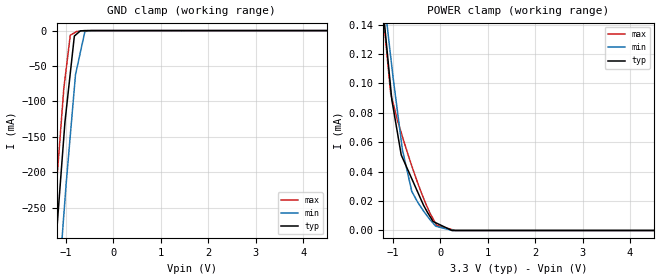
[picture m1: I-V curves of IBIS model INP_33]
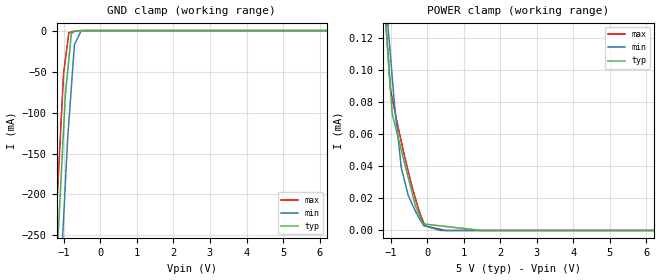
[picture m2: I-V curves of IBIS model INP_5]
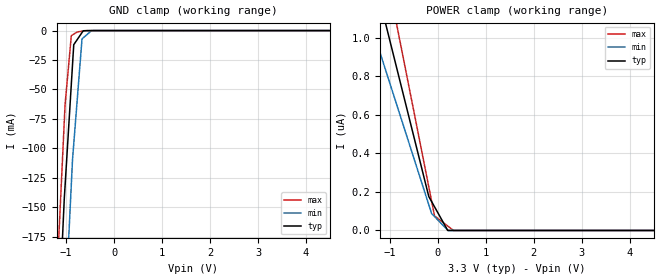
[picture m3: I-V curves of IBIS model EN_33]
| Texas Instruments Incorporated
| 6KVpeak Low Power Triple and Quad Channels Digital Isolators
| 25 Mbps (C) and 150 Mbps (M) speed grades.
| Marketing part#   Voltage Range   Package-type   #pins/pkg drawing
| ISO7640FMDW   3V - 5.5V   SOIC   16-pin DW
| ISO7640FMDWR   3V - 5.5V   SOIC   16-pin DW
| ISO7640FCDW   3V - 5.5V   SOIC   16-pin DW
| ISO7640FCDWR   3V - 5.5V   SOIC   16-pin DW
| ISO7641FMDW   3V - 5.5V   SOIC   16-pin DW
| ISO7641FMDWR   3V - 5.5V   SOIC   16-pin DW
| ISO7641FCDW   3V - 5.5V   SOIC   16-pin DW
| ISO7641FCDWR   3V - 5.5V   SOIC   16-pin DW
| ISO7631FMDW   3V - 5.5V   SOIC   16-pin DW
| ISO7631FMDWR   3V - 5.5V   SOIC   16-pin DW
| ISO7631FCDW   3V - 5.5V   SOIC   16-pin DW
| ISO7631FCDWR   3V - 5.5V   SOIC   16-pin DW
[IBIS Ver]   4.0
[File name]   iso75xx.ibs
[File Rev]   1.1
[Date]   03/13/2012
[Source]   Model built from TISPICED simulations at:
   Texas Instruments Incorporated.
   Analog-eLab, HPA
   12500 TI Blvd
   Dallas, TX -75243
   For Support e-mail: elab_ibis@list.ti.com
[Notes]   Revision History
   Rev 1.0: 6/13/2011
   Rev 1.1: 3/13/2012 Added 25 Mbps speed grade output buffer
   - Pulldown/up in OUTM/OUTC non-monotonic warnings reflect true buffer behavior
   - C_comp although listed in numberical order of value are obtained from varying PVT conditions.
   For PVT conditions for each specific value, refer to the buffer description under repective [Model].
   IBIS model user is responsible for using appropriate C_comp to simulate for Signal Integrity.
[Disclaimer] This model is designed as an aid for customers of Texas Instruments.
 TI and its licensors and suppliers make no warranties, either expressed
 or implied, with respect to this  model, including the warranties of
 merchantability or fitness for a particular purpose.
 The model is provided solely on an "as is" basis. The entire risk as to
 its quality and performance is with the customer.
[Copyright] (C)Copyright 2012 Texas Instruments Incorporated.
   All rights reserved.
|   Component ISO7640F
[Component]   ISO7640F
[Manufacturer]  Texas Instruments Incorporated
[Package]   |16-pin SOIC DW package
|   typ   min   max
R_pkg   0.10903   0.02188   0.19738
L_pkg   1.81763nH   0.55719nH   2.72701nH
C_pkg   0.46541pF   0.23901pF   0.75876pF
[Pin] signal_name   model_name   R_pin   L_pin   C_pin
   1  VCC1   POWER   0.10139   2.72701n   0.70015p
   2  GND1   GND   0.12533   2.59840n   0.28313p
   3  INA   INP   0.19738   2.59444n   0.23901p
   4  INB   INP   0.12501   1.60826n   0.59739p
   5  INC   INP   0.09868   1.27583n   0.33612p
   6  IND   INP   0.15228   1.98345n   0.42023p
   7  NC   NC   0.02188   0.55719n   0.33803p
   8  GND1   GND   0.09581   2.52990n   0.46538p
   9  GND2   GND   0.10168   2.16452n   0.38933p
   10  EN   EN   0.16987   2.23387n   0.49303p
   11  OUTD   OUT   0.14297   1.85926n   0.49369p
   12  OUTC   OUT   0.10283   1.32835n   0.29474p
   13  OUTB   OUT   0.07399   1.10755n   0.43265p
   14  OUTA   OUT   0.08416   1.26268n   0.45009p
   15  GND2   GND   0.06629   1.45518n   0.75876p
   16  VCC2   POWER   0.08496   1.80603n   0.75490p
[Pin Mapping]pulldown_ref pullup_ref gnd_clamp_ref power_clamp_ref |ext_ref
1   NC   PWRBUS1  |VCC1
2   GNDBUS1   NC   |GND1
3   NC   NC   GNDBUS1   PWRBUS1
4   NC   NC   GNDBUS1   PWRBUS1
5   NC   NC   GNDBUS1   PWRBUS1
6   NC   NC   GNDBUS1   PWRBUS1
7   NC   NC
8   GNDBUS1   NC   |GND1
9   GNDBUS2   NC   |GND2
10   NC   NC   GNDBUS2   PWRBUS2
11   GNDBUS2   PWRBUS2   GNDBUS2   PWRBUS2
12   GNDBUS2   PWRBUS2   GNDBUS2   PWRBUS2
13   GNDBUS2   PWRBUS2   GNDBUS2   PWRBUS2
14   GNDBUS2   PWRBUS2   GNDBUS2   PWRBUS2
15   GNDBUS2   NC   |GND2
16   NC   PWRBUS2  |VCC2
|   Component ISO7641F
[Component]   ISO7641F
[Manufacturer]  Texas Instruments Incorporated
[Package]   |16-pin SOIC DW package
|   typ   min   max
R_pkg   0.10681   0.06298   0.16885
L_pkg   1.70911nH   1.15087nH   2.22009nH
C_pkg   0.45120pF   0.20111pF   0.73257pF
[Pin] signal_name   model_name   R_pin   L_pin   C_pin
   1  VCC1   POWER   0.08793   2.21738n   0.66791p
   2  GND1   GND   0.10467   2.09455n   0.25132p
   3  INA   INP   0.13798   1.78864n   0.20111p
   4  INB   INP   0.09011   1.16823n   0.57349p
   5  INC   INP   0.10921   1.41023n   0.34068p
   6  OUTD   OUT   0.14555   1.89355n   0.41488p
   7  EN1   EN   0.16885   2.22009n   0.43190p
   8  GND1   GND   0.08161   2.08117n   0.43691p
   9  GND2   GND   0.07697   1.92728n   0.40234p
   10  EN2   EN   0.15712   2.06097n   0.48728p
   11  IND   INP   0.11312   1.46878n   0.47723p
   12  OUTC   OUT   0.10925   1.41018n   0.29792p
   13  OUTB   OUT   0.10585   1.36324n   0.34974p
   14  OUTA   OUT   0.07689   1.15087n   0.42179p
   15  GND2   GND   0.06298   1.36962n   0.73218p
   16  VCC2   POWER   0.08085   1.72105n   0.73257p
[Pin Mapping]pulldown_ref pullup_ref gnd_clamp_ref power_clamp_ref |ext_ref
1   NC   PWRBUS1  |VCC1
2   GNDBUS1   NC   |GND1
3   NC   NC   GNDBUS1   PWRBUS1
4   NC   NC   GNDBUS1   PWRBUS1
5   NC   NC   GNDBUS1   PWRBUS1
6   GNDBUS1   PWRBUS1   GNDBUS1   PWRBUS1
7   NC   NC   GNDBUS1   PWRBUS1
8   GNDBUS1   NC   |GND1
9   GNDBUS2   NC   |GND2
10   NC   NC   GNDBUS2   PWRBUS2
11   NC   NC   GNDBUS2   PWRBUS2
12   GNDBUS2   PWRBUS2   GNDBUS2   PWRBUS2
13   GNDBUS2   PWRBUS2   GNDBUS2   PWRBUS2
14   GNDBUS2   PWRBUS2   GNDBUS2   PWRBUS2
15   GNDBUS2   NC   |GND2
16   NC   PWRBUS2  |VCC2
|   Component ISO7631F
[Component]   ISO7631F
[Manufacturer]  Texas Instruments Incorporated
[Package]   |16-pin SOIC DW package
|   typ   min   max
R_pkg   0.10681   0.06298   0.16885
L_pkg   1.70911nH   1.15087nH   2.22009nH
C_pkg   0.45120pF   0.20111pF   0.73257pF
[Pin] signal_name   model_name   R_pin   L_pin   C_pin
   1  VCC1   POWER   0.08793   2.21738n   0.66791p
   2  GND1   GND   0.10467   2.09455n   0.25132p
   3  INA   INP   0.13798   1.78864n   0.20111p
   4  INB   INP   0.09011   1.16823n   0.57349p
   5  OUTC   OUT   0.10921   1.41023n   0.34068p
   6  NC   NC   0.14555   1.89355n   0.41488p
   7  EN1   EN   0.16885   2.22009n   0.43190p
   8  GND1   GND   0.08161   2.08117n   0.43691p
   9  GND2   GND   0.07697   1.92728n   0.40234p
   10  EN2   EN   0.15712   2.06097n   0.48728p
   11  NC   NC   0.11312   1.46878n   0.47723p
   12  INC   INP   0.10925   1.41018n   0.29792p
   13  OUTB   OUT   0.10585   1.36324n   0.34974p
   14  OUTA   OUT   0.07689   1.15087n   0.42179p
   15  GND2   GND   0.06298   1.36962n   0.73218p
   16  VCC2   POWER   0.08085   1.72105n   0.73257p
[Pin Mapping]pulldown_ref pullup_ref gnd_clamp_ref power_clamp_ref |ext_ref
1   NC   PWRBUS1  |VCC1
2   GNDBUS1   NC   |GND1
3   NC   NC   GNDBUS1   PWRBUS1
4   NC   NC   GNDBUS1   PWRBUS1
5   GNDBUS1   PWRBUS1   GNDBUS1   PWRBUS1
6   NC   NC   NC   NC
7   NC   NC   GNDBUS1   PWRBUS1
8   GNDBUS1   NC   |GND1
9   GNDBUS2   NC   |GND2
10   NC   NC   GNDBUS2   PWRBUS2
11   NC   NC
12   NC   NC   GNDBUS2   PWRBUS2
13   GNDBUS2   PWRBUS2   GNDBUS2   PWRBUS2
14   GNDBUS2   PWRBUS2   GNDBUS2   PWRBUS2
15   GNDBUS2   NC   |GND2
16   NC   PWRBUS2  |VCC2
[Model Selector] INP
INP_33   INP Input model for 3.0V - 3.6V
INP_5   INP Input model for 4.5V - 5.5V
[Model Selector] EN
EN_33   EN Input model for 3.0V - 3.6V
EN_5   EN Input model for 4.5V - 5.5V
[Model Selector] OUT
OUTM_33   Output model for 3.0V - 3.6V, 150 Mbps max datarate
OUTM_5   Output model for 4.5V - 5.5V, 150 Mbps max datarate
OUTC_33   Output model for 3.0V - 3.6V, 25 Mbps max datarate
OUTC_5   Output model for 4.5V - 5.5V, 25 Mbps max datarate
| Models and submodels in the file (8): INP_33 (Input), INP_5 (Input), EN_33 (Input), EN_5 (Input), OUTM_33 (3-state), OUTM_5 (3-state), OUTC_5 (3-state), OUTC_33 (3-state)
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|   INP_33 Model
[Model]   INP_33
Model_type   Input
Vinl = .8
Vinh = 2
|   typ   min   max
|   (typ PVT)   (Fast PVT)   (Slow PVT)
C_comp   0.4547p   0.3924p   0.5244p
[Voltage Range]   3.3   3   3.6
[Temperature Range]   27   125   -40
[Power Clamp Reference]   3.3   3   3.6
[GND Clamp Reference]   -0   -0   -0
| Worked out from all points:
|   GND clamp passes 1 mA (typ) near -0.71 V on its own axis
[GND Clamp]
|   Voltage   I(typ)   I(min)   I(max)
-3.3V     -2.332A    -2.436A    -2.268A
-1.394V   -467.7mA   -579.5mA   -397.5mA
-1.244V   -327.2mA   -439.7mA   -256.1mA
-1.196V   -283.3mA   -394.7mA   -213.7mA
-1.046V   -150.4mA   -260.4mA   -81.66mA
-909.8mV  -60.2mA    -148.2mA   -6.478mA
-824.2mV  -7.726mA   -81.21mA   -3.179mA
-800mV    -6.326mA   -62.34mA   -2.25mA
-773.4mV  -4.78mA    -54.13mA   -1.224mA
-602mV    -88.69uA   -1.316mA   -137.7uA
-475.9mV  -46.02uA   -55.21uA   -12.29uA
6.6V      0A         0A         0A
[POWER Clamp]
|   Voltage   I(typ)   I(min)   I(max)
-3.3V     952uA      800.7uA    1.137mA
-1.196V   146.8uA    160.4uA    143.7uA
-1.046V   96.81uA    118.1uA    92.98uA
-1.022V   88.8uA     111.4uA    89.92uA
-824.2mV  51.34uA    61.14uA    66.48uA
-800mV    49.59uA    55.12uA    63.91uA
-602mV    35.2uA     26.59uA    43.91uA
-355.6mV  17.3uA     13.32uA    22.1uA
-152.1mV  6.109uA    4.946uA    7.838uA
-97.62mV  5.269uA    2.928uA    4.583uA
243.9mV   0A         96.16nA    640.9nA
6.6V      0A         0A         0A
|   INP_5 Model
[Model]   INP_5
Model_type   Input
Vinl = .8
Vinh = 2
|   typ   min   max
|   (typ PVT)   (Fast PVT)   (Slow PVT)
C_comp   0.4382p   0.3816p   0.5008p
[Voltage Range]   5   4.5   5.5
[Temperature Range]   27   125   -40
[Power Clamp Reference]   5   4.5   5.5
[GND Clamp Reference]   -0   -0   -0
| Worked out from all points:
|   GND clamp passes 1 mA (typ) near -0.71 V on its own axis
|   POWER clamp passes 1 mA (typ) near -3.42 V on its own axis
[GND Clamp]
|   Voltage   I(typ)   I(min)   I(max)
-5V       -4.018A    -4.118A    -3.957A
-1.259V   -340.9mA   -454.1mA   -273mA
-1.197V   -286.5mA   -395.6mA   -218.4mA
-1.008V   -121.3mA   -230mA     -52.5mA
-959.3mV  -79.09mA   -187.6mA   -35.8mA
-897mV    -50.58mA   -133.1mA   -14.28mA
-863.3mV  -35.2mA    -112.3mA   -2.661mA
-793.7mV  -3.338mA   -69.1mA    -1.734mA
-709.7mV  -1.113mA   -17.05mA   -688.5uA
-522.4mV  -167.4uA   -172.5uA   -35.62uA
10V       0A         0A         0A
[POWER Clamp]
|   Voltage   I(typ)   I(min)   I(max)
-5V       1.594mA    1.312mA    1.93mA
-1.197V   149.3uA    161.3uA    151.2uA
-1.008V   88.33uA    109.2uA    88.16uA
-959.3mV  72.74uA    95.91uA    82.61uA
-897mV    67.11uA    78.77uA    75.45uA
-709.7mV  50.18uA    39.01uA    55.39uA
-522.4mV  33.26uA    22.04uA    37.06uA
-335.3mV  16.35uA    12.67uA    20.89uA
-99.29mV  4.077uA    3.044uA    4.866uA
488.3mV   2.557uA    0A         0A
1.477V    0A         0A         0A
10V       0A         0A         0A
|   EN_33 Model
[Model]   EN_33
Model_type   Input
Vinl = .8
Vinh = 2
|   typ   min   max
|   (typ PVT)   (Fast PVT)   (Slow PVT)
C_comp   0.4547p   0.3924p   0.5244p
[Voltage Range]   3.3   3   3.6
[Temperature Range]   27   125   -40
[Power Clamp Reference]   3.3   3   3.6
[GND Clamp Reference]   -0   -0   -0
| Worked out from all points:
|   GND clamp passes 1 mA (typ) near -0.66 V on its own axis
[GND Clamp]
|   Voltage   I(typ)   I(min)   I(max)
-3.3V     -2.332A    -2.436A    -2.268A
-1.22V    -305.3mA   -417.7mA   -234mA
-1.065V   -166.3mA   -275.8mA   -99.86mA
-1.039V   -143.3mA   -254.2mA   -77.66mA
-1.022V   -132.1mA   -240.1mA   -63.17mA
-891.8mV  -45.59mA   -130.6mA   -4.244mA
-866.8mV  -29.04mA   -109.6mA   -3.643mA
-841.1mV  -11.98mA   -96.29mA   -3.023mA
-761.3mV  -7.216mA   -54.96mA   -1.1mA
-668.8mV  -1.695mA   -7.086mA   -556.6uA
-470.8mV  -6.873uA   -45.96uA   -12.71uA
6.6V      0A         0A         0A
[POWER Clamp]
|   Voltage   I(typ)   I(min)   I(max)
-3.3V     3.293uA    2.564uA    4.156uA
-1.616V   1.601uA    1.243uA    2.024uA
-643.1mV  629.7nA    486.8nA    798.6nA
-188.8mV  176.3nA    133.7nA    226.5nA
-130mV    150nA      87.95nA    152.4nA
-68.86mV  122.7nA    72.19nA    75.43nA
206.1mV   0A         1.323nA    23.05nA
327.1mV   0A         0A         0A
6.6V      0A         0A         0A
